| TEXAS INSTRUMENTS INCORPORATED
| Standard Linear and Logic Group
| IBIS Model of SN74AHCT125
| QUADRUPLE BUS BUFFER GATES WITH 3-STATE OUTPUTS
| This file contains package information for the following:
|  PDIP 14-pin (N) package as [Component] AHCT125A_N
|  SOIC 14-pin (D) package as [Component] AHCT125A_D
|  SSOP 14-pin (DB) package as [Component] AHCT125A_DB
|  TVSOP 14-pin (DGV) package as [Component] AHCT125A_DGV
|  SOP 14-pin (NS) package as [Component] AHCT125A_NS
|  TSSOP 14-pin (PW) package as [Component] AHCT125A_PW
|  QFN 14-pin (RGY) package as [Component] AHCT125A_RGY
| This device can be powered at the following Vccs:
|  5 volt Vcc
| This file provides unique models under the [Model Selector] for each Vcc.
| For operation at a specific Vcc, select the appropriate model after each
| [Model Selector] keyword.
[IBIS Ver]   3.2
[Comment char]  |_char
[File Name]   sn74ahct125.ibs
[File Rev]   1.1 | b_die
[Date]   March 3, 2006
[Source]   Data created from TI-SPICE simulations at TI-SLL.
[Notes]   The following is an IBIS list for the AHCT125A.
   Please contact sllibis@ti.com with questions and
   comments concerning SLL IBIS models.
   - FILE REV HISTORY
   - 1.1 Release IBIS file on 03/09/06
   - C_comp values are taken at a different test condition
   than the data sheet.
   - As there is no power clamp diode in the IN and NOE
   Models, we removed the Power Clamp table data from those
   Models.
[Disclaimer] Property of Texas Instruments Incorporated.  Unauthorized
   reproduction and/or distribution is strictly prohibited.
   This product is protected under copyright law.
   Created  2006, (C) Copyright  2006, Texas Instruments
   Incorporated, All Rights Reserved
   UNLESS THERE IS A SIGNED, WRITTEN AGREEMENT TO THE
   CONTRARY, TEXAS INSTRUMENTS (TI) IS PROVIDING THE IBIS
   MODELS  AND WITHOUT ANY WARRANTY, EXPRESSED OR
   IMPLIED.  TI assumes no liability for:
   1) the accuracy of the IBIS models provided to your
   company;
   2) the proper functioning of these IBIS Models in your
   design or for any resulting applications; or
   3) infringement of patents, copyrights or intellectual
   property rights resulting from your use of these IBIS
   models.
   TI provides IBIS Models as a service to our customers.
   You and your company shall not distribute, sell or give
   these models to anyone else without prior written
   permission from TI.
   TI reserves the right to make changes to our products or
   to discontinue any semiconductor product or service
   without notice, and advises our customers to obtain the
   latest version of relevant information to verify, before
   placing orders, that the information being relied on is
   current.
   Please be aware that your receipt and use of the IBIS
   information provided shall serve as acceptance of these
   terms and conditions.  If you do not accept these terms,
   you should return or destroy the IBIS models and any
   other accompanying information immediately.
| Component AHCT125A_N 14-pin PDIP
[Component]   AHCT125A_N
[Manufacturer]   Texas Instruments, Inc.
[Package]
|   typ   min   max
R_pkg   4.500e-02   3.700e-02   6.300e-02
L_pkg   5.407e-09   3.922e-09   6.942e-09
C_pkg   3.890e-13   2.050e-13   6.040e-13
[Pin]   signal_name   model_name   R_pin   L_pin   C_pin
1   1NOE   AHCT125_NOE   6.300e-02   6.942e-09   6.040e-13
2   1A   AHCT125_IN   3.700e-02   6.200e-09   4.060e-13
3   1Y   AHCT125_OUT   4.200e-02   4.389e-09   3.220e-13
4   2NOE   AHCT125_NOE   3.800e-02   3.922e-09   2.050e-13
5   2A   AHCT125_IN   3.900e-02   4.301e-09   2.980e-13
6   2Y   AHCT125_OUT   3.800e-02   5.329e-09   3.560e-13
7   GND   GND   5.300e-02   6.510e-09   5.440e-13
8   3Y   AHCT125_OUT   5.300e-02   6.437e-09   5.390e-13
9   3A   AHCT125_IN   3.900e-02   5.352e-09   3.470e-13
10   3NOE   AHCT125_NOE   4.200e-02   4.473e-09   2.970e-13
11   4Y   AHCT125_OUT   4.400e-02   4.326e-09   2.250e-13
12   4A   AHCT125_IN   4.200e-02   4.295e-09   2.800e-13
13   4NOE   AHCT125_NOE   4.200e-02   6.318e-09   4.180e-13
14   VCC   POWER   6.100e-02   6.900e-09   6.030e-13
| Component AHCT125A_D 14-pin SOIC
[Component]   AHCT125A_D
[Manufacturer]   Texas Instruments, Inc.
[Package]
|   typ   min   max
R_pkg   3.100e-02   2.800e-02   3.400e-02
L_pkg   3.109e-09   2.462e-09   3.889e-09
C_pkg   4.730e-13   3.630e-13   6.280e-13
[Pin]   signal_name   model_name   R_pin   L_pin   C_pin
1   1NOE   AHCT125_NOE   3.300e-02   3.854e-09   6.220e-13
2   1A   AHCT125_IN   3.200e-02   3.188e-09   4.730e-13
3   1Y   AHCT125_OUT   2.800e-02   2.462e-09   3.770e-13
4   2NOE   AHCT125_NOE   3.100e-02   2.596e-09   3.630e-13
5   2A   AHCT125_IN   2.800e-02   2.521e-09   3.720e-13
6   2Y   AHCT125_OUT   3.400e-02   3.250e-09   4.760e-13
7   GND   GND   3.400e-02   3.889e-09   6.280e-13
8   3Y   AHCT125_OUT   3.400e-02   3.889e-09   6.280e-13
9   3A   AHCT125_IN   3.400e-02   3.250e-09   4.760e-13
10   3NOE   AHCT125_NOE   2.800e-02   2.521e-09   3.720e-13
11   4Y   AHCT125_OUT   3.100e-02   2.596e-09   3.640e-13
12   4A   AHCT125_IN   2.800e-02   2.462e-09   3.770e-13
13   4NOE   AHCT125_NOE   3.200e-02   3.188e-09   4.730e-13
14   VCC   POWER   3.300e-02   3.854e-09   6.220e-13
| Component AHCT125A_DB 14-pin SSOP
[Component]   AHCT125A_DB
[Manufacturer]   Texas Instruments, Inc.
[Package]
|   typ   min   max
R_pkg   4.400e-02   4.100e-02   4.600e-02
L_pkg   3.551e-09   3.258e-09   3.927e-09
C_pkg   4.020e-13   3.600e-13   4.210e-13
[Pin]   signal_name   model_name   R_pin   L_pin   C_pin
1   1NOE   AHCT125_NOE   4.600e-02   3.927e-09   4.080e-13
2   1A   AHCT125_IN   4.400e-02   3.587e-09   4.210e-13
3   1Y   AHCT125_OUT   4.100e-02   3.289e-09   3.980e-13
4   2NOE   AHCT125_NOE   4.200e-02   3.258e-09   3.600e-13
5   2A   AHCT125_IN   4.100e-02   3.286e-09   4.030e-13
6   2Y   AHCT125_OUT   4.400e-02   3.586e-09   4.210e-13
7   GND   GND   4.600e-02   3.927e-09   4.080e-13
8   3Y   AHCT125_OUT   4.600e-02   3.927e-09   4.080e-13
9   3A   AHCT125_IN   4.400e-02   3.586e-09   4.210e-13
10   3NOE   AHCT125_NOE   4.100e-02   3.286e-09   4.030e-13
11   4Y   AHCT125_OUT   4.300e-02   3.258e-09   3.600e-13
12   4A   AHCT125_IN   4.100e-02   3.289e-09   3.980e-13
13   4NOE   AHCT125_NOE   4.400e-02   3.587e-09   4.210e-13
14   VCC   POWER   4.600e-02   3.927e-09   4.080e-13
| Component AHCT125A_DGV 14-pin TVSOP
[Component]   AHCT125A_DGV
[Manufacturer]   Texas Instruments, Inc.
[Package]
|   typ   min   max
R_pkg   3.500e-02   2.000e-02   4.500e-02
L_pkg   2.499e-09   2.077e-09   2.966e-09
C_pkg   3.610e-13   3.050e-13   4.160e-13
[Pin]   signal_name   model_name   R_pin   L_pin   C_pin
1   1NOE   AHCT125_NOE   2.700e-02   2.717e-09   3.730e-13
2   1A   AHCT125_IN   3.700e-02   2.434e-09   3.980e-13
3   1Y   AHCT125_OUT   3.400e-02   2.200e-09   3.160e-13
4   2NOE   AHCT125_NOE   2.000e-02   2.077e-09   3.090e-13
5   2A   AHCT125_IN   3.000e-02   2.147e-09   3.050e-13
6   2Y   AHCT125_OUT   4.200e-02   2.580e-09   4.080e-13
7   GND   GND   3.900e-02   2.921e-09   3.850e-13
8   3Y   AHCT125_OUT   3.300e-02   2.841e-09   3.800e-13
9   3A   AHCT125_IN   4.200e-02   2.611e-09   4.100e-13
10   3NOE   AHCT125_NOE   3.800e-02   2.331e-09   3.290e-13
11   4Y   AHCT125_OUT   2.600e-02   2.223e-09   3.190e-13
12   4A   AHCT125_IN   3.400e-02   2.259e-09   3.130e-13
13   4NOE   AHCT125_NOE   4.500e-02   2.681e-09   4.160e-13
14   VCC   POWER   4.200e-02   2.966e-09   3.860e-13
| Component AHCT125A_NS 14-pin SOP
[Component]   AHCT125A_NS
[Manufacturer]   Texas Instruments, Inc.
[Package]
|   typ   min   max
R_pkg   4.500e-02   3.900e-02   5.400e-02
L_pkg   3.796e-09   2.561e-09   4.952e-09
C_pkg   5.280e-13   2.880e-13   7.100e-13
[Pin]   signal_name   model_name   R_pin   L_pin   C_pin
1   1NOE   AHCT125_NOE   4.700e-02   4.867e-09   7.060e-13
2   1A   AHCT125_IN   5.100e-02   4.083e-09   5.920e-13
3   1Y   AHCT125_OUT   4.100e-02   2.915e-09   3.760e-13
4   2NOE   AHCT125_NOE   3.900e-02   2.561e-09   2.880e-13
5   2A   AHCT125_IN   4.100e-02   3.101e-09   4.300e-13
6   2Y   AHCT125_OUT   4.700e-02   4.047e-09   5.890e-13
7   GND   GND   5.100e-02   4.909e-09   7.000e-13
8   3Y   AHCT125_OUT   4.500e-02   4.784e-09   6.940e-13
9   3A   AHCT125_IN   5.400e-02   4.176e-09   5.970e-13
10   3NOE   AHCT125_NOE   3.900e-02   3.287e-09   4.490e-13
11   4Y   AHCT125_OUT   3.900e-02   2.586e-09   2.940e-13
12   4A   AHCT125_IN   4.000e-02   2.802e-09   3.710e-13
13   4NOE   AHCT125_NOE   4.900e-02   4.080e-09   5.930e-13
14   VCC   POWER   5.200e-02   4.952e-09   7.100e-13
| Component AHCT125A_PW 14-pin TSSOP
[Component]   AHCT125A_PW
[Manufacturer]   Texas Instruments, Inc.
[Package]
|   typ   min   max
R_pkg   3.200e-02   2.900e-02   3.500e-02
L_pkg   2.378e-09   2.170e-09   2.680e-09
C_pkg   3.140e-13   2.700e-13   3.350e-13
[Pin]   signal_name   model_name   R_pin   L_pin   C_pin
1   1NOE   AHCT125_NOE   3.300e-02   2.618e-09   3.300e-13
2   1A   AHCT125_IN   3.100e-02   2.313e-09   3.170e-13
3   1Y   AHCT125_OUT   3.000e-02   2.310e-09   3.140e-13
4   2NOE   AHCT125_NOE   3.100e-02   2.173e-09   2.720e-13
5   2A   AHCT125_IN   3.000e-02   2.204e-09   3.090e-13
6   2Y   AHCT125_OUT   3.200e-02   2.315e-09   3.170e-13
7   GND   GND   3.500e-02   2.680e-09   3.350e-13
8   3Y   AHCT125_OUT   3.300e-02   2.640e-09   3.330e-13
9   3A   AHCT125_IN   3.400e-02   2.347e-09   3.190e-13
10   3NOE   AHCT125_NOE   2.900e-02   2.277e-09   3.130e-13
11   4Y   AHCT125_OUT   3.100e-02   2.170e-09   2.700e-13
12   4A   AHCT125_IN   3.100e-02   2.244e-09   3.110e-13
13   4NOE   AHCT125_NOE   3.300e-02   2.343e-09   3.210e-13
14   VCC   POWER   3.500e-02   2.657e-09   3.320e-13
| Component AHCT125A_RGY 14-pin QFN
[Component]   AHCT125A_RGY
[Manufacturer]   Texas Instruments, Inc.
[Package]
|   typ   min   max
R_pkg   3.300e-02   3.000e-02   3.500e-02
L_pkg   7.380e-10   6.850e-10   7.840e-10
C_pkg   3.160e-13   3.040e-13   3.230e-13
[Pin]   signal_name   model_name   R_pin   L_pin   C_pin
1   1NOE   AHCT125_NOE   3.500e-02   7.840e-10   3.040e-13
2   1A   AHCT125_IN   3.400e-02   7.690e-10   3.160e-13
3   1Y   AHCT125_OUT   3.300e-02   7.360e-10   3.210e-13
4   2NOE   AHCT125_NOE   3.300e-02   7.390e-10   3.170e-13
5   2A   AHCT125_IN   3.100e-02   6.910e-10   3.170e-13
6   2Y   AHCT125_OUT   3.100e-02   6.970e-10   3.180e-13
7   GND   GND   3.200e-02   7.130e-10   3.160e-13
8   3Y   AHCT125_OUT   3.500e-02   7.830e-10   3.120e-13
9   3A   AHCT125_IN   3.400e-02   7.680e-10   3.150e-13
10   3NOE   AHCT125_NOE   3.400e-02   7.720e-10   3.230e-13
11   4Y   AHCT125_OUT   3.300e-02   7.340e-10   3.170e-13
12   4A   AHCT125_IN   3.000e-02   6.880e-10   3.150e-13
13   4NOE   AHCT125_NOE   3.000e-02   6.850e-10   3.150e-13
14   VCC   POWER   3.400e-02   7.730e-10   3.130e-13
| Models and submodels in the file (3): AHCT125_IN (Input), AHCT125_NOE (Input), AHCT125_OUT (3-state)
